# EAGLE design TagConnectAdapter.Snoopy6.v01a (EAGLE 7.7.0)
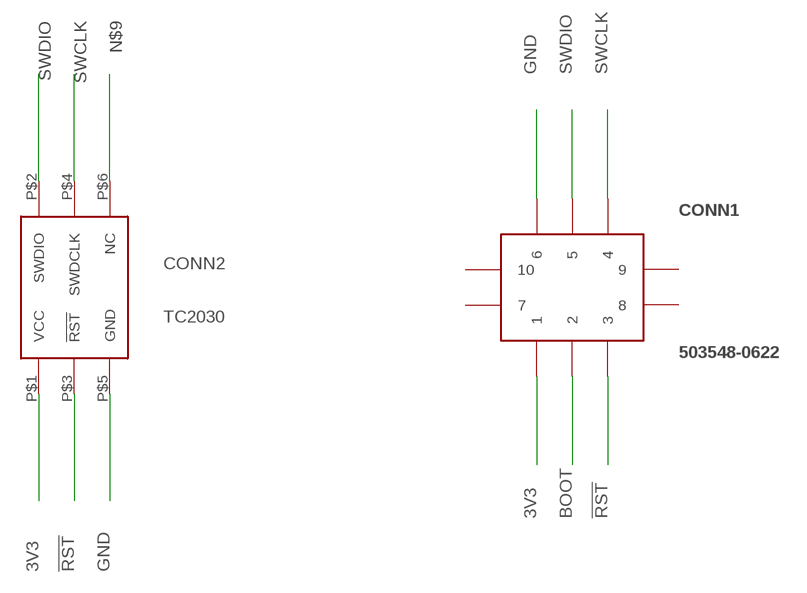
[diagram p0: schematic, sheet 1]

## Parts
CONN1  503548-0622  [503548-0622]
CONN2  TC2030  [TC2030]

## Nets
3V3: CONN1.P$1 CONN2.P$1(VCC)
!RST: CONN1.P$3 CONN2.P$3(!RST)
BOOT: CONN1.P$2
GND: CONN1.P$6 CONN2.P$5(GND)
N$9: CONN2.P$6(NC)
SWCLK: CONN1.P$4 CONN2.P$4(SWDCLK)
SWDIO: CONN1.P$5 CONN2.P$2(SWDIO)
Unconnected: CONN1.P$7 CONN1.P$8 CONN1.P$9 CONN1.P$10

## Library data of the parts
CONN1 = kris:503548-0622: 503548-0622 Molex low-profile male connector https://www.molex.com/pdm_docs/sd/5035480622_sd.pdf
CONN2 = kris:TC2030: TC2030 SWD pogo pin contact pad

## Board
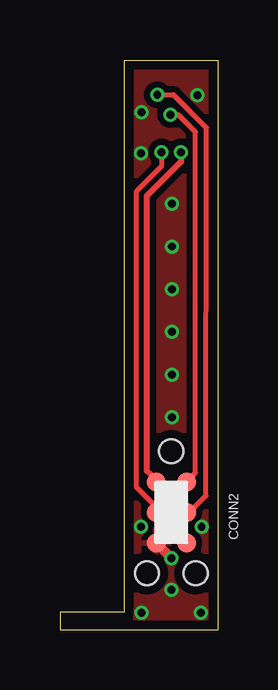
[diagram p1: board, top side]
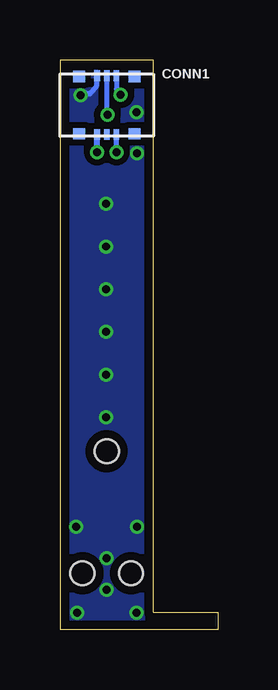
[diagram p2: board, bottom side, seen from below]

Size 6.6 x 23.75 mm. Coordinates in mm from the lower left corner, seen from the top.
Outline: 0,0 6.6,0 6.6,23.75 2.69,23.75 2.69,0.74 0,0.74 0,0
Copper layers (1*16): Top 0.035559375mm / dielectric 1.6mm / Bottom 0.035559375mm
Design rules "oshpark-2layer *": minimum track width 6mil, minimum drill 10mil, track to track 6mil, track to pad 6mil, pad to pad 6mil, via to via 6mil, smd to smd 6mil, copper to edge 15mil, drill to drill 6mil, minimum pad ring 5mil, minimum via ring 5mil, stop-mask expansion 2.5mil, vias tented up to drill 20mil, thermal gap 10mil

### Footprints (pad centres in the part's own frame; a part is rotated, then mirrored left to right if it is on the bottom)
503548-0622 = smd 0.24 x 0.45: P$1 -0.4,-1.225; P$2 0,-1.225; P$3 0.4,-1.225; P$4 0.4,1.225; P$5 0,1.225; P$6 -0.4,1.225 | smd 0.5 x 0.47: P$7 -1.15,-1.195; P$8 1.15,-1.195; P$9 1.15,1.195; P$10 -1.15,1.195
TC2030 = smd 0.787 x 0.787: P$1 -1.27,-0.635; P$2 -1.27,0.635; P$3 0,-0.635; P$4 0,0.635; P$5 1.27,-0.635; P$6 1.27,0.635 | hole 0.991: -2.54,0; 2.54,1.016; 2.54,-1.016

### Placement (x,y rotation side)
CONN1  4.65,21.87 0 bottom
CONN2  4.65,4.9 270 top

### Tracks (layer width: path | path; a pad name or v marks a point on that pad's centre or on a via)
3V3  (via drill 0.33)
  Top 0.254: CONN2.P$1 4.01,6.3 3.63,6.63 3.63,18.09 5.05,19.51 v5.05,19.91
  Bottom 0.254: v5.05,19.91 CONN1.P$1
!RST  (via drill 0.33)
  Top 0.203: CONN2.P$3 4.01,5.13 3.2,5.94 3.2,18.29 4.24,19.33 v4.24,19.91
  Bottom 0.203: v4.24,19.91 CONN1.P$3
GND  (via drill 0.33)
  Top 0.406: CONN2.P$5 v4.65,3
  Bottom 0.203: CONN1.P$6 5.07,22.66 5.36,22.35
  Bottom 0.254: 5.36,22.35 v5.74,22.28
  other vias: 3.4,21.56 3.38,19.86 3.4,0.71 5.89,0.71 4.65,1.68 3.38,4.29 5.92,4.29 4.67,17.75 4.67,15.98 4.67,14.2 4.67,12.42 4.67,10.64 4.67,8.86
  pour Top (isolate 0.254): 2.69,23.75 6.6,23.75 6.6,0 2.69,0
  pour Bottom (isolate 0.254): 2.69,23.75 6.6,23.75 6.6,0 2.69,0
SWCLK  (via drill 0.33)
  Top 0.203: CONN2.P$4 5.41,4.9 6.1,5.59 6.12,20.93 4.75,22.3 v4.06,22.3
  Bottom 0.203: CONN1.P$4 4.25,22.54 v4.06,22.3
SWDIO  (via drill 0.33)
  Top 0.203: CONN2.P$2 5.66,6.55 5.66,20.75 4.95,21.46 v4.62,21.46
  Bottom 0.203: CONN1.P$5 4.65,21.49 v4.62,21.46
